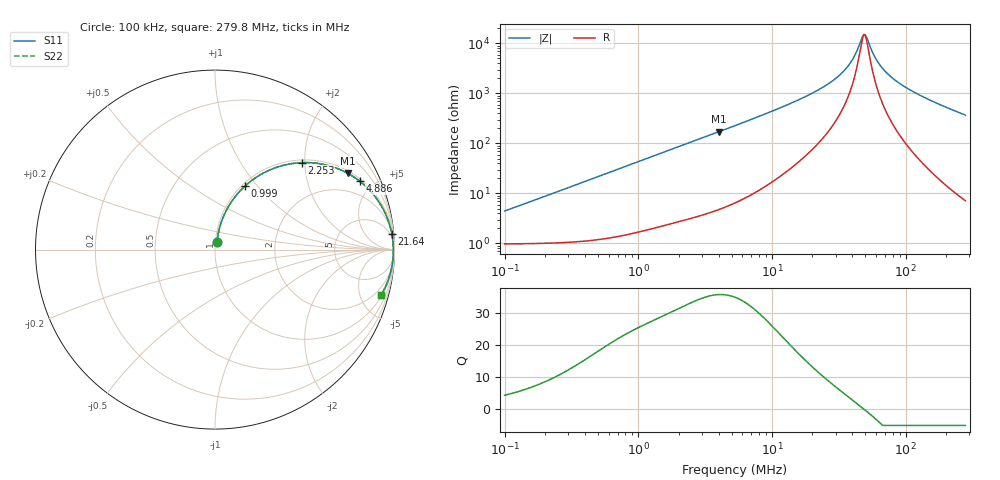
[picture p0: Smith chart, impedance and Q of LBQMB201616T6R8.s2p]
! LBQMB201616T6R8  S-PARAMETER MODEL  ( General Type )
! Model Generated by TAIYO YUDEN Corporation (http://www.ty-top.com)
! Version 1.0
! TAIYO YUDEN Control No. 191025NI43SB-FBB
! Copyright(c) 2019 TAIYO YUDEN CO.,LTD. All Rights Reserved.
! Product Description (link to TY-COMPAS)
! https://ds.yuden.co.jp/TYCOMPAS/or/detail?pn=LBQMB201616T6R8J&u=M
! Products Name : Inductors
! Characteristics :
!  Inductance : 6.8 uH , SRF(min) : 33 MHz , DC Resistance(max) : 1.261 Ohm , Rated Current : 240 mA
!  Case Size : 2.0 x 1.6 / 0.079 x 0.063 [mm/inch] , Thickness : 1.6 / 0.063 [mm/inch]
!  (Conditions: Temperature = 25 degC , DC Bias Current/Voltage = 0A / 0V)
! External Node Assignments :
!  1  o---GGG---o  2
! GND o---------o GND
! Frequency Range : 0.1MHz  -  279.750408MHz  [ 402 STEP ]
# MHz S RI R 50
! Freq[MHz].  S11 Real  S11 Imag  S21 Real  S21 Imag  S12 Real  S12 Imag  S22 Real  S22 Imag
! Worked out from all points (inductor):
!   401 points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, 100 kHz to 279.8 MHz, reference 50 ohm
!   read as one part in series: L = 6.93 uH near 104 kHz
!   highest Q = 35.9 at 4.006 MHz (marker M1), where L = 6.8 uH
!   self-resonance near 48.81 MHz
!   S11 on the Smith chart (normalised r, x): 100 kHz: 1.02, +0.09; 999 kHz: 1.03, +0.86; 2.253 MHz: 1.06, +1.93; 4.886 MHz: 1.12, +4.18; 21.64 MHz: 3, +23; 279.8 MHz: 1.14, -7.35
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0.1  0.0115 0.0426  0.9885 -0.0426  0.9885 -0.0426  0.0115 0.0426
0.377863  0.0363 0.1566  0.9637 -0.1566  0.9637 -0.1566  0.0363 0.1566
0.998995  0.1665 0.3535  0.8335 -0.3535  0.8335 -0.3535  0.1665 0.3535
1.427803  0.2806 0.4322  0.7194 -0.4322  0.7194 -0.4322  0.2806 0.4322
2.2535  0.4821 0.4845  0.5179 -0.4845  0.5179 -0.4845  0.4821 0.4845
4.006345  0.7397 0.4251  0.2603 -0.4251  0.2603 -0.4251  0.7397 0.4251
4.885597  0.8072 0.3807  0.1928 -0.3807  0.1928 -0.3807  0.8072 0.3807
5.289144  0.8302 0.3615  0.1698 -0.3615  0.1698 -0.3615  0.8302 0.3615
9.21848  0.9349 0.2292  0.0651 -0.2292  0.0651 -0.2292  0.9349 0.2292
19.9857  0.9832 0.0964  0.0168 -0.0964  0.0168 -0.0964  0.9832 0.0964
21.63651  0.9852 0.0862  0.0148 -0.0862  0.0148 -0.0862  0.9852 0.0862
28.56434  0.99 0.054  0.00998 -0.054  0.00998 -0.054  0.99 0.054
35.53124  0.9922 0.0313  0.00785 -0.0313  0.00785 -0.0313  0.9922 0.0313
40.82525  0.9929 0.0177  0.00705 -0.0177  0.00705 -0.0177  0.9929 0.0177
46.90804  0.9934 0.00437  0.00662 -0.00437  0.00662 -0.00437  0.9934 0.00437
48.80689  0.9934 0.000574  0.00656 -0.000574  0.00656 -0.000574  0.9934 0.000574
50.78261  0.9935 -0.00322  0.00653 0.00322  0.00653 0.00322  0.9935 -0.00322
57.20271  0.9934 -0.0147  0.0066 0.0147  0.0066 0.0147  0.9934 -0.0147
61.92761  0.9932 -0.0224  0.0068 0.0224  0.0068 0.0224  0.9932 -0.0224
75.51853  0.9921 -0.0426  0.00786 0.0426  0.00786 0.0426  0.9921 -0.0426
124.0157  0.984 -0.102  0.016 0.102  0.016 0.102  0.984 -0.102
279.7504  0.9269 -0.2507  0.0731 0.2507  0.0731 0.2507  0.9269 -0.2507
